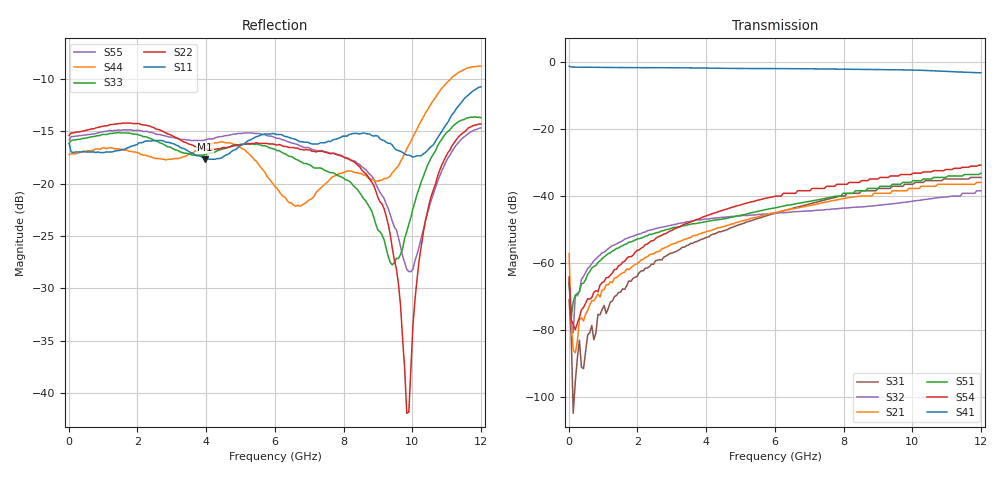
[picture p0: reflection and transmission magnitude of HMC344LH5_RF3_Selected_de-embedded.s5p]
! Hittite Microwave Corporation
! 20 Alpha Road
! Chelmsford, MA 01824
! Tel: 978-250-3343
! Fax: 978-250-3373
! Device: HMC344LH5, DC-12 GHz GaAs MMIC SP4T Non-Reflective Switch in Hermetic Leadless SMT Package
! Misc: Data was de-embedded to package pins.
!  Port 1 = RFC
!  Port 2 = RF1
!  Port 3 = RF2
!  Port 4 = RF3
!  Port 5 = RF4
!  RF3 selected, Vctl= 0/-5 V
!  Data reformated to new Touchstone file format - Tue Jan 09 13:46:17  2007
# MHz S DB R 50
! 5 Port Network Data
! freq  dbS11  angS11  dbS12  angS12  dbS13  angS13  dbS14  angS14
!  dbS15  angS15
!  dbS21  angS21  dbS22  angS22  dbS23  angS23
!  dbS24  angS24  dbS25  angS25
!  dbS31  angS31  dbS32  angS32
!  dbS33  angS33  dbS34  angS34  dbS35  angS35
!  dbS41  angS41
!  dbS42  angS42  dbS43  angS43  dbS44  angS44  dbS45  angS45
!  dbS51  angS51  dbS52  angS52  dbS53  angS53  dbS54  angS54
!  dbS55  angS55
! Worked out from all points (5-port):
!   201 points, 10 MHz to 12 GHz, reference 50 ohm
!   strongest paths, dB at 10 MHz, 3.007 GHz, 6.005 GHz, 9.002 GHz, 12 GHz:
!     S41: -1.1, -1.6, -1.9, -2.2, -3.1
!     S54: -64.2, -50.2, -40.1, -34.9, -30.8
!     S51: -65.9, -49.6, -43.5, -37.7, -33.2
!     S21: -57.2, -54.4, -45.0, -39.2, -35.9
!     S32: -64.9, -48.7, -45.1, -42.8, -38.4
!     S31: -71.0, -57.0, -45.2, -37.7, -34.4
!   lowest |S11| = -17.7 dB at 3.967 GHz (marker M1), VSWR 1.30, Z = 42.5 - j9.57 ohm
!   |S11| at or under -10 dB: start of sweep to end of sweep
